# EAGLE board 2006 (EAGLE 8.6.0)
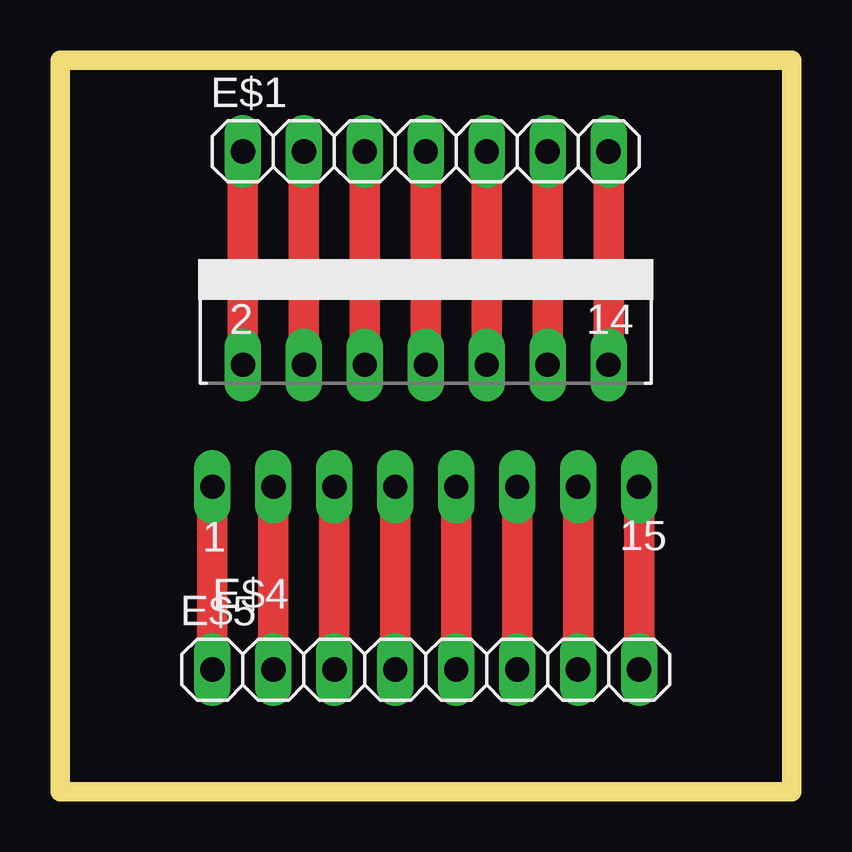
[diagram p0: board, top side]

Size 30.48 x 30.48 mm. Coordinates in mm from the lower left corner, seen from the top.
Outline: 0,30.48 30.48,30.48 30.48,0 0,0 0,30.48
Copper layers (1*16): Top 0.035mm / dielectric 1.5mm / Bottom 0.035mm
Design rules "default": minimum track width 6mil, minimum drill 0.35mm, track to track 6mil, track to pad 6mil, pad to pad 6mil, via to via 6mil, smd to smd 6mil, copper to edge 40mil, drill to drill 6mil, minimum pad ring 10mil, minimum via ring 8mil, stop-mask expansion 4mil, vias tented up to drill 0mil, thermal gap 10mil

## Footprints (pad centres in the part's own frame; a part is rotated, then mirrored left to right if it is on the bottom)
1X07 = drill 1.016 long: 1 -7.62,0; 2 -5.08,0; 3 -2.54,0; 4 0,0; 5 2.54,0; 6 5.08,0; 7 7.62,0
MULTIWATT-15 = drill 1.016 long: 1 -8.89,-7.62; 2 -7.62,-2.54; 3 -6.35,-7.62; 4 -5.08,-2.54; 5 -3.81,-7.62; 6 -2.54,-2.54; 7 -1.27,-7.62; 8 0,-2.54; 9 1.27,-7.62; 10 2.54,-2.54; 11 3.81,-7.62; 12 5.08,-2.54; 13 6.35,-7.62; 14 7.62,-2.54; 15 8.89,-7.62
1X08 = drill 1.016 long: 1 -8.89,0; 2 -6.35,0; 3 -3.81,0; 4 -1.27,0; 5 1.27,0; 6 3.81,0; 7 6.35,0; 8 8.89,0

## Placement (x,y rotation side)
E$1  [1X07]  15.24,26.67 0 top
E$4  [MULTIWATT-15]  15.24,20.32 0 top
E$5  [1X08]  15.24,5.08 0 top

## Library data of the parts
E$1 E$5 = pinhead
E$4 = ref-packages

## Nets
S$1: E$4.15 E$5.8
S$2: E$4.13 E$5.7
S$3: E$4.11 E$5.6
S$4: E$4.9 E$5.5
S$5: E$4.7 E$5.4
S$6: E$4.5 E$5.3
S$7: E$4.3 E$5.2
S$8: E$4.1 E$5.1
S$9: E$1.7 E$4.14
S$10: E$1.6 E$4.12
S$11: E$1.5 E$4.10
S$12: E$1.4 E$4.8
S$13: E$1.3 E$4.6
S$14: E$1.2 E$4.4
S$15: E$1.1 E$4.2

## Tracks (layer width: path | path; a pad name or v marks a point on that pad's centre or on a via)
S$1
  Top 1.27: E$5.8 E$4.15
S$2
  Top 1.27: E$5.7 E$4.13
S$3
  Top 1.27: E$5.6 E$4.11
S$4
  Top 1.27: E$5.5 E$4.9
S$5
  Top 1.27: E$5.4 E$4.7
S$6
  Top 1.27: E$5.3 E$4.5
S$7
  Top 1.27: E$5.2 E$4.3
S$8
  Top 1.27: E$5.1 E$4.1
S$9
  Top 1.27: E$4.14 E$1.7
S$10
  Top 1.27: E$4.12 E$1.6
S$11
  Top 1.27: E$4.10 E$1.5
S$12
  Top 1.27: E$4.8 E$1.4
S$13
  Top 1.27: E$4.6 E$1.3
S$14
  Top 1.27: E$4.4 E$1.2
S$15
  Top 1.27: E$4.2 E$1.1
